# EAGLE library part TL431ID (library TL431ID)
2% Accuracy Adjustable Precision Shunt Regulator Source: Datasheet
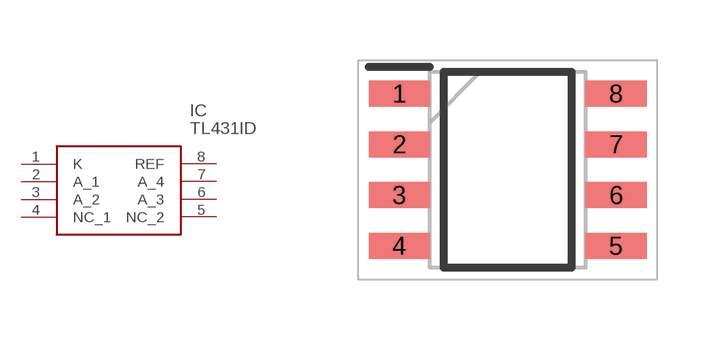
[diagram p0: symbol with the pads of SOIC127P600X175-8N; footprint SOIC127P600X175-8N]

Designator prefix IC

## TL431ID (Description: 2% Accuracy Adjustable Precision Shunt Regulator; Height: 1.75mm; Manufacturer_Name: Texas Instruments; Manufacturer_Part_Number: TL431ID; Mouser_Part_Number: 595-TL431ID; Mouser_Price-Stock: https://www.mouser.co.uk/ProductDetail/Texas-Instruments/TL431ID?qs=8Pd2FuFSoMGOQLhJS1fgeg%3D%3D)  [SOIC127P600X175-8N]
1  K
2  A_1
3  A_2
4  NC_1
5  NC_2
6  A_3
7  A_4
8  REF

## Footprint SOIC127P600X175-8N (pad centres in mm)
D0008A
smd 1.528 x 0.65: 1 -2.711,1.905; 2 -2.711,0.635; 3 -2.711,-0.635; 4 -2.711,-1.905; 5 2.711,-1.905; 6 2.711,-0.635; 7 2.711,0.635; 8 2.711,1.905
